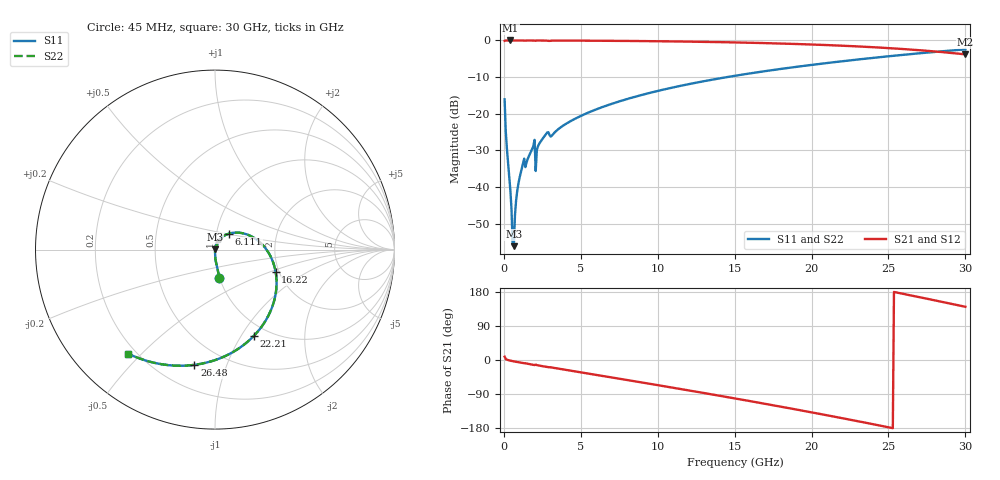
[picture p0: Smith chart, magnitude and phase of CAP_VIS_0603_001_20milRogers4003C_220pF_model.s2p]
! S-parameter model data by Modelithics Inc.  support@modelithics.com  813-866-6335  Tampa FL USA
! S-Parameter data specifications:
! Substrate: 20-mil Rogers 4003C, substrate thickness, H=0.508mm, Dielectric constant, Er=3.75
! PCB Mounting Pad Footprint: Pad width, PadW=0.90mm , Pad length, PadL=1.00mm , Pad gap, PadG (edge-to-edge)=1.00mm , Reference planes=3.0mm apart
! Created Wed Nov 18 13:33:10 2015
# hz S ma R 50
! 2 Port Network Data from SP1.SP block
! freq  magS11  angS11  magS21  angS21  magS12  angS12  magS22  angS22
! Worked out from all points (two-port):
!   401 points, 45 MHz to 30 GHz, reference 50 ohm
!   highest |S21| = 0.00 dB at 419.4 MHz (marker M1); lowest = -3.8 dB at 30 GHz (marker M2)
!   |S21| within 3 dB of the highest: start of sweep to 28.02 GHz
!   lowest |S11| = -56.1 dB at 644.1 MHz (marker M3), VSWR 1.00, Z = 50.1 + j0.141 ohm
!   |S11| at or under -10 dB: start of sweep to 14.49 GHz
!   |S22| runs from -56.1 to -2.4 dB; largest |S21 - S12| = 0
!   S11 on the Smith chart (normalised r, x): 45 MHz: 1.00, -0.32; 6.111 GHz: 1.15, +0.21; 16.22 GHz: 1.92, -0.56; 22.21 GHz: 0.86, -1.14; 26.48 GHz: 0.35, -0.78; 30 GHz: 0.17, -0.46
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4.5e7  0.1576 -81.1  0.9873 8.8  0.9873 8.8  0.1576 -81.1
1.94775e8  0.03326 -88.5  0.9991 0.8  0.9991 0.8  0.03326 -88.5
4.194375e8  0.009027 -88.6  0.9994 -1.8  0.9994 -1.8  0.009027 -88.6
4.94325e8  0.004957 -86.3  0.9994 -2.4  0.9994 -2.4  0.004957 -86.3
6.441e8  0.00157 63.9  0.9993 -3.6  0.9993 -3.6  0.00157 63.9
7.189875e8  0.004177 77.1  0.9993 -4.2  0.9993 -4.2  0.004177 77.1
9.4365e8  0.01123 80.4  0.9991 -5.8  0.9991 -5.8  0.01123 80.4
1.168312e9  0.01816 79.1  0.9986 -7.4  0.9986 -7.4  0.01816 79.1
1.8423e9  0.03327 75.9  0.998 -12.0  0.998 -12.0  0.03327 75.9
2.216738e9  0.03622 73.7  0.9978 -14.2  0.9978 -14.2  0.03622 73.7
2.291625e9  0.03895 73.3  0.9977 -14.7  0.9977 -14.7  0.03895 73.3
2.74095e9  0.05314 67.7  0.9944 -18.0  0.9944 -18.0  0.05314 67.7
5.062462e9  0.09491 55.9  0.9934 -33.1  0.9934 -33.1  0.09491 55.9
6.110888e9  0.1173 49.1  0.9908 -40.0  0.9908 -40.0  0.1173 49.1
1.007992e10  0.2069 22.5  0.9752 -66.9  0.9752 -66.9  0.2069 22.5
1.50225e10  0.3299 -11.9  0.9398 -101.5  0.9398 -101.5  0.3299 -11.9
1.62207e10  0.3614 -20.6  0.9279 -110.1  0.9279 -110.1  0.3614 -20.6
2.003996e10  0.4652 -48.9  0.8797 -138.5  0.8797 -138.5  0.4652 -48.9
2.22117e10  0.5267 -65.6  0.8439 -155.2  0.8439 -155.2  0.5267 -65.6
2.505742e10  0.6099 -88.4  0.7852 -178.0  0.7852 -178.0  0.6099 -88.4
2.648029e10  0.6522 -100.1  0.7502 170.3  0.7502 170.3  0.6522 -100.1
3e10  0.7552 -129.9  0.6458 140.4  0.6458 140.4  0.7552 -129.9
